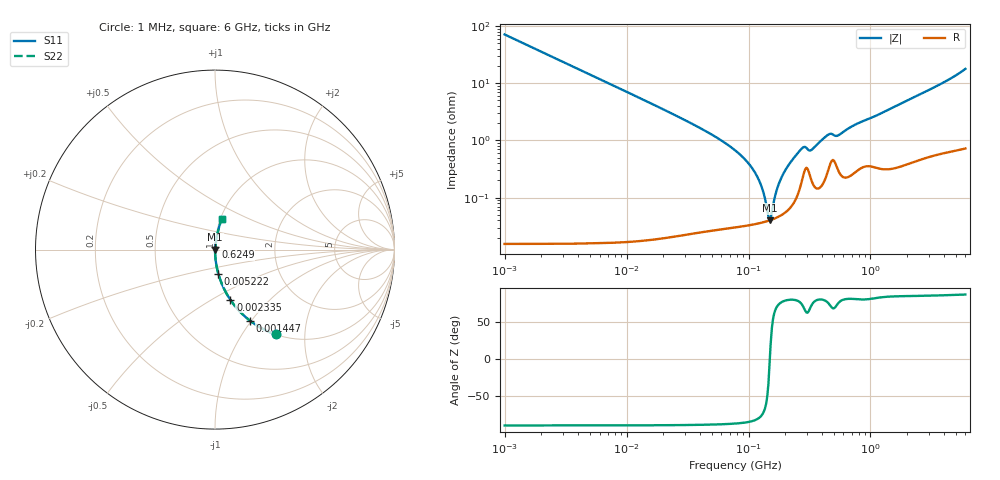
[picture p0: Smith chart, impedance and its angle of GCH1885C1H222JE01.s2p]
!Murata Part Number: GCH1885C1H222JE01
!These Parameters are Measured in Series Mode Connection
!Data Generated on Mar 13, 2026
!  o--ll--o
!Port1  Port2
!  o------o
!Operation Temp=25[degC], DC Bias Voltage=0[V]
!Freq. Start=1000[kHz] Stop=6[GHz] 401[Steps]
# Hz S RI R 50
!Freq.(Hz) S11(Real) S11(Imag) S21(Real) S21(Imag) S12(Real) S12(Imag) S22(Real) S22(Imag)
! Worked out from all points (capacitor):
!   401 points, 1 MHz to 6 GHz, reference 50 ohm
!   read as one part in series: C = 2.23 nF near 1.044 MHz
!   lowest |Z| = 40.3 mohm at 148.7 MHz (marker M1)
!   series resonance near 149.5 MHz, so ESL is about 510 pH
!   S11 on the Smith chart (normalised r, x): 1 MHz: 1.00, -1.43; 1.447 MHz: 1.00, -0.99; 2.335 MHz: 1.00, -0.61; 5.222 MHz: 1.00, -0.27; 624.9 MHz: 1.00, +0.03; 6 GHz: 1.01, +0.36
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1000000  0.3371 -0.4726  0.6629 0.4726  0.6629 0.4726  0.3371 -0.4726
1447343  0.1954 -0.3963  0.8046 0.3963  0.8046 0.3963  0.1954 -0.3963
2335446  0.0854 -0.2792  0.9146 0.2792  0.9146 0.2792  0.0854 -0.2792
4293785  0.0269 -0.1614  0.9731 0.1614  0.9731 0.1614  0.0269 -0.1614
5222143  0.0184 -0.1338  0.9816 0.1338  0.9816 0.1338  0.0184 -0.1338
1.843659e7  0.00163 -0.038  0.9984 0.038  0.9984 0.038  0.00163 -0.038
7.745967e7  0.000346 -0.00673  0.9997 0.00673  0.9997 0.00673  0.000346 -0.00673
9.83954e7  0.000342 -0.00412  0.9997 0.00412  0.9997 0.00412  0.000342 -0.00412
1.170949e8  0.000355 -0.00237  0.9996 0.00237  0.9996 0.00237  0.000355 -0.00237
1.305463e8  0.00037 -0.00131  0.9996 0.00131  0.9996 0.00131  0.00037 -0.00131
1.424119e8  0.000388 -0.000472  0.9996 0.000472  0.9996 0.000472  0.000388 -0.000472
1.487431e8  0.0004 -5.03e-05  0.9996 5.03e-05  0.9996 5.03e-05  0.0004 -5.03e-05
1.553559e8  0.000413 0.000373  0.9996 -0.000373  0.9996 -0.000373  0.000413 0.000373
1.770109e8  0.000469 0.00167  0.9995 -0.00167  0.9995 -0.00167  0.000469 0.00167
2.061188e8  0.000589 0.00329  0.9994 -0.00329  0.9994 -0.00329  0.000589 0.00329
2.734687e8  0.00199 0.00695  0.998 -0.00695  0.998 -0.00695  0.00199 0.00695
3.325952e8  0.00189 0.00671  0.9981 -0.00671  0.9981 -0.00671  0.00189 0.00671
4.509737e8  0.00319 0.0122  0.9968 -0.0122  0.9968 -0.0122  0.00319 0.0122
5.366786e8  0.00331 0.0116  0.9967 -0.0116  0.9967 -0.0116  0.00331 0.0116
6.249308e8  0.00245 0.0148  0.9975 -0.0148  0.9975 -0.0148  0.00245 0.0148
1.428092e9  0.00435 0.0348  0.9957 -0.0348  0.9957 -0.0348  0.00435 0.0348
6e9  0.0374 0.1706  0.9626 -0.1706  0.9626 -0.1706  0.0374 0.1706
